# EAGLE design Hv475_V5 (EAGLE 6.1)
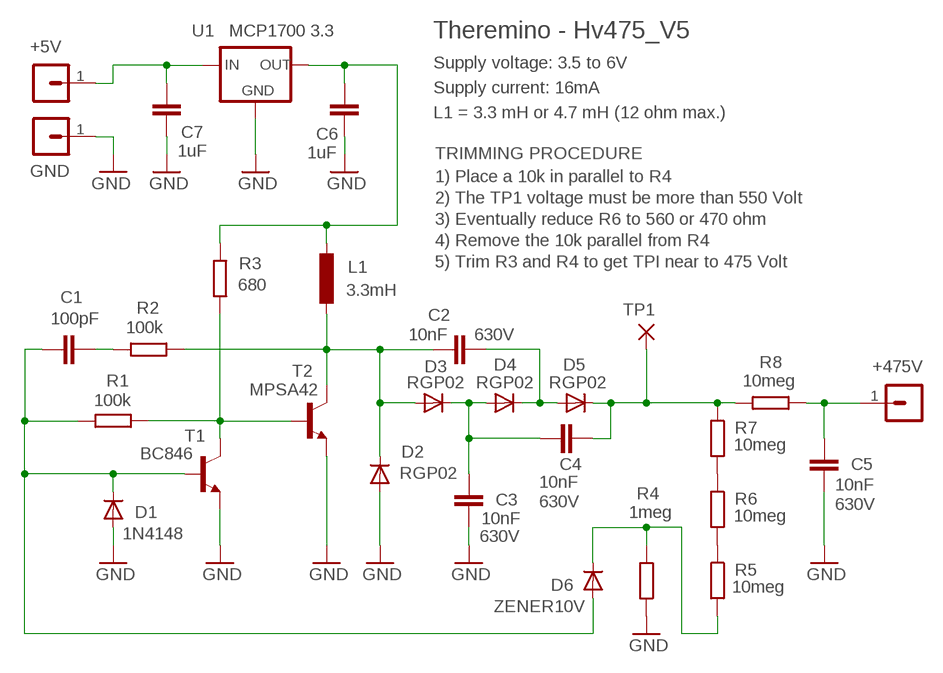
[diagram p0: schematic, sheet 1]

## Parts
+5V  MA01-1  [MA01-1]
+475V  MA01-1  [MA01-1]
C1  100pF  C-EU025-024X044  [C025-024X044]
C2  10nF  C-EU050-024X044  [C050-024X044]
C3  10nF  C-EU050-024X044  [C050-024X044]
C4  10nF  C-EU050-024X044  [C050-024X044]
C5  10nF  C-EU050-024X044  [C050-024X044]
C6  1uF  C-EUC0805  [C0805]
C7  1uF  C-EUC0805  [C0805]
D1  1N4148  DIODE-DO34-7  [DO34-7]
D2  RGP02  DIODE-DO34-7  [DO34-7]
D3  RGP02  DIODE-DO34-7  [DO34-7]
D4  RGP02  DIODE-DO34-7  [DO34-7]
D5  RGP02  DIODE-DO34-7  [DO34-7]
D6  ZENER10V  DIODE-DO34-7  [DO34-7]
GND  MA01-1  [MA01-1]
L1  3.3mH  INDUCTORL_VERT_508  [L_VERT_508]
R1  100k  R-EU_0204/7  [0204/7]
R2  100k  R-EU_0204/7  [0204/7]
R3  680  R-EU_0204/7  [0204/7]
R4  1meg  R-EU_0204/7  [0204/7]
R5  10meg  R-EU_0204/7  [0204/7]
R6  10meg  R-EU_0204/7  [0204/7]
R7  10meg  R-EU_0204/7  [0204/7]
R8  10meg  R-EU_0204/7  [0204/7]
T1  BC846  -NPN-TO92-CBE  [TO92-CBE]
T2  MPSA42  -NPN-TO92-EBC  [TO92-EBC]
TP1  TEST  WIREPAD1,6/0,8  [1,6/0,8]
U1  MCP1700 3.3  MCP1700L1  [TO92L1]

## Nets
+5V: C6.1 L1.+ R3.2 U1.1(OUT)
GND: C3.1 C5.1 C6.2 C7.2 D1.A D2.A GND.1 R4.1 T1.E T2.E U1.3(GND)
N$1: D6.C R4.2 R5.2
N$2: C1.2 R2.2
N$3: R5.1 R6.2
N$4: C1.1 D1.C D6.A R1.2 T1.B
N$5: C4.2 D5.C R7.1 R8.2 TP1.1(P)
N$6: C2.1 D2.C D3.A L1.- R2.1 T2.C
N$7: +5V.1 C7.1 U1.2(IN)
N$8: R6.1 R7.2
N$11: C3.2 C4.1 D3.C D4.A
N$15: +475V.1 C5.2 R8.1
N$17: C2.2 D4.C D5.A
N$26: R1.1 R3.1 T1.C T2.B

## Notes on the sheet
- Theremino - Hv475_V5
- Supply voltage: 3.5 to 6V
- Supply current: 16mA
- L1 = 3.3 mH or 4.7 mH (12 ohm max.)
- TRIMMING PROCEDURE
- 1) Place a 10k in parallel to R4
- 2) The TP1 voltage must be more than 550 Volt
- 3) Eventually reduce R6 to 560 or 470 ohm
- 4) Remove the 10k parallel from R4
- 5) Trim R3 and R4 to get TPI near to 475 Volt

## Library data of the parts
+5V +475V GND = 03-con-lstb-M:MA01-1: PIN HEADER
C1 C6 C7 = 00-LIVIO:C-EU: CAPACITOR, European symbol
C2-C5 = 00-LIVIO:C-EU: CAPACITOR, European symbol; VOLTAGE: 630V
D1-D6 = 00-LIVIO:DIODE-: DIODE
L1 = 00-LIVIO:INDUCTOR
R1-R8 = 00-LIVIO:R-EU_: RESISTOR, European symbol
T1 T2 = 00-LIVIO:*-NPN-: NPN Transistror
TP1 = 00-LIVIO:WIREPAD: Wire PAD connect wire on PCB
U1 = 00-LIVIO:MCP1700: Linear regulator Quescient courrent 1.8uA Input 2.3v to 6v Output 1.2v 1.8v 2.5v 3.0v 3.3v 5.0v

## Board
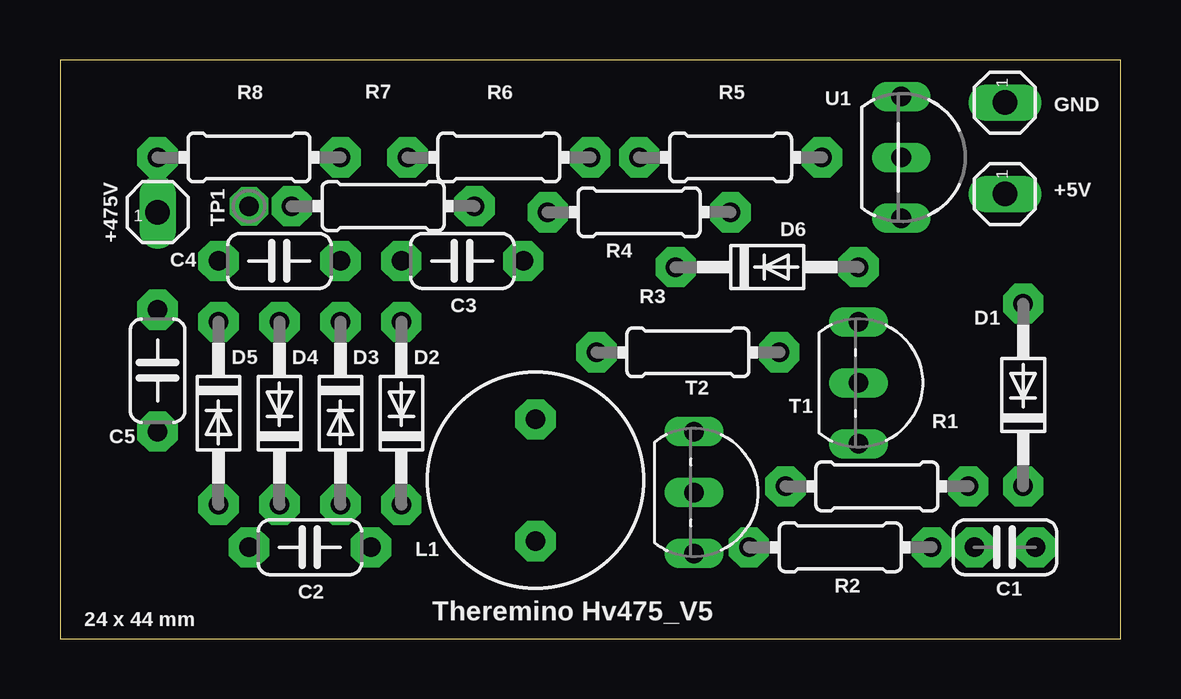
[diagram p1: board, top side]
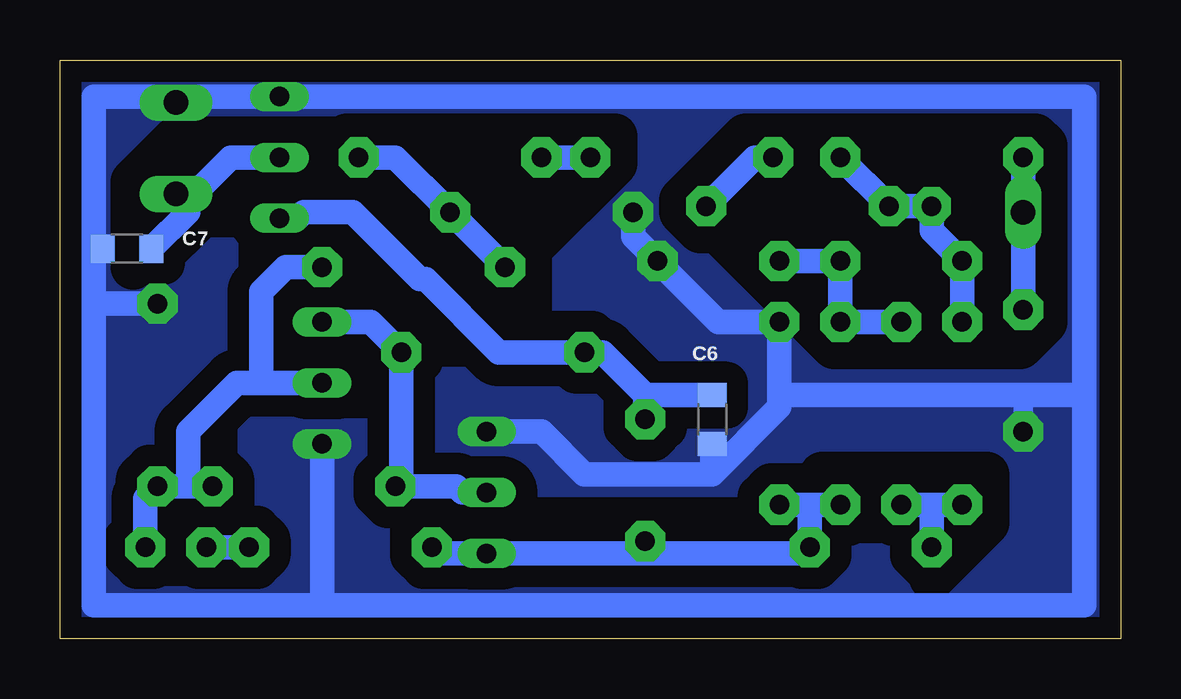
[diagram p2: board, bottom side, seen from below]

Size 44.2 x 24.13 mm. Coordinates in mm from the lower left corner, seen from the top.
Outline: 0,0 44.2,0 44.2,24.13 0,24.13 0,0
Copper layers (1*16): Top 0.035mm / dielectric 1.5mm / Bottom 0.035mm
Design rules: minimum track width 10mil, minimum drill 31mil, track to track 31mil, track to pad 31mil, pad to pad 31mil, via to via 31mil, smd to smd 31mil, copper to edge 31mil, drill to drill 8mil, minimum pad ring 5mil, minimum via ring 8mil, stop-mask expansion 4mil, vias tented up to drill 0mil, thermal gap 47mil
bRestrict: 22 lines

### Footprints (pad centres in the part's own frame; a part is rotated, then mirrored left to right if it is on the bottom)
MA01-1 = drill 1.016 long: 1 0,0
C025-024X044 = drill 0.813 pad 1.676 octagon: 1 -1.27,0; 2 1.27,0
C050-024X044 = drill 0.813 pad 1.676 octagon: 1 -2.54,0; 2 2.54,0
C0805 = smd 1 x 1.2: 1 -1.016,0; 2 1.016,0
DO34-7 = drill 0.813 pad 1.676 octagon: A 3.81,0; C -3.81,0
L_VERT_508 = drill 0.813 pad 1.676 octagon: + -2.54,0; - 2.54,0
0204/7 = drill 0.813 pad 1.676 octagon: 1 -3.81,0; 2 3.81,0
TO92-CBE = drill 0.813 long: B 0,0; C -2.54,0; E 2.54,0
TO92-EBC = drill 0.813 long: B 0,0; C 2.54,0; E -2.54,0
1,6/0,8 = drill 0.813 pad 1.6 octagon: 1 0,0
TO92L1 = drill 0.813 long: 1 2.54,0; 2 0,0; 3 -2.54,0

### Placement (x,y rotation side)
+5V  39.37,18.54 270 top
+475V  4.06,17.78 0 top
C1  39.37,3.81 180 top
C2  10.41,3.81 180 top
C3  16.76,15.75 180 top
C4  9.14,15.75 180 top
C5  4.06,11.18 90 top
C6  17.02,9.14 270 bottom
C7  41.4,16.26 180 bottom
D1  40.13,10.16 90 top
D2  14.22,9.4 90 top
D3  11.68,9.4 270 top
D4  9.14,9.4 90 top
D5  6.6,9.4 270 top
D6  29.46,15.49 0 top
GND  39.37,22.35 270 top
L1  19.81,6.6 270 top
R1  34.04,6.35 0 top
R2  32.51,3.81 0 top
R3  26.16,11.94 180 top
R4  24.13,17.78 0 top
R5  27.94,20.07 0 top
R6  18.29,20.07 0 top
R7  13.46,18.03 0 top
R8  7.87,20.07 0 top
T1  33.27,10.67 270 top
T2  26.42,6.1 270 top
TP1  7.87,18.03 180 top
U1  35.05,20.07 270 top

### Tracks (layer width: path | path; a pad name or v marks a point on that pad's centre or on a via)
+5V
  Bottom 1.016: 19.81,10.16 21.59,11.94 R3.2 25.91,11.94 28.96,14.99 29.21,14.99 32,17.78 34.04,17.78 34.29,17.53 U1.1 | L1.+ 19.81,10.16 | 19.81,10.16 C6.1
GND
  Bottom 0.813: C5.1 4.06,10.16
  Bottom 1.016: 17.02,6.86 22.35,6.86 24.13,8.64 T2.E | 17.02,6.86 14.22,9.65 14.22,10.16 | 14.22,10.16 4.06,10.16 1.52,10.16 | 33.27,1.4 1.52,1.4 1.52,10.16 | 33.27,1.4 42.8,1.4 42.8,13.97 | 42.8,16.26 42.8,22.61 39.37,22.61 | 39.37,22.61 U1.3 1.52,22.61 1.52,10.16 | T1.E 33.27,1.4 | R4.1 20.32,16.76 C3.1 16.76,13.21 D2.A 14.22,10.16 | D1.A 42.8,13.97 | C6.2 17.02,6.86 | GND.1 39.37,22.61 | 42.8,13.97 42.8,16.26 | 42.8,16.26 C7.2
  pour Bottom (isolate 0.9, rank 6, no thermals): -1,-1 45.2,-1 45.2,25.13 -1,25.13
N$1
  Bottom 1.016: 31.24,20.07 R5.2 30.23,20.07 R4.2 D6.C
N$2
  Bottom 1.016: R2.2 C1.2
N$3
  Bottom 1.016: R6.2 R5.1
N$4
  Bottom 1.016: C1.1 40.64,5.84 D1.C 38.86,6.35 | 38.86,6.35 R1.2 | 35.81,10.67 36.83,10.67 38.86,8.64 38.86,6.35 | T1.B 35.81,10.67 | 35.81,10.67 35.81,14.48 34.8,15.49 D6.A
N$5
  Bottom 1.016: D5.C C4.2 7.87,17.02 TP1.1 R7.1 R8.2
N$6
  Bottom 1.016: 19.81,3.56 12.95,3.56 C2.1 12.95,5.59 D2.C D3.A | 19.81,3.56 L1.- | 19.81,3.56 T2.C 28.7,3.56 R2.1
N$7
  Bottom 1.016: 38.86,18.54 38.61,18.54 37.08,20.07 U1.2 | C7.1 38.86,17.78 38.86,18.54 | 38.86,18.54 +5V.1
N$8
  Bottom 1.016: R6.1 15.24,20.07 R7.2
N$11
  Bottom 1.016: C3.2 C4.1 D3.C D4.A
N$15
  Bottom 1.016: R8.1 +475V.1 C5.2
N$17
  Bottom 1.016: C2.2 7.87,5.59 D4.C D5.A
N$26
  Bottom 1.016: T2.B 27.43,6.1 27.69,6.35 29.97,6.35 | R1.1 29.97,6.35 | T1.C 31.24,13.21 R3.1 29.97,6.35

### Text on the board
tNames: 24 x 44 mm | Theremino Hv475_V5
